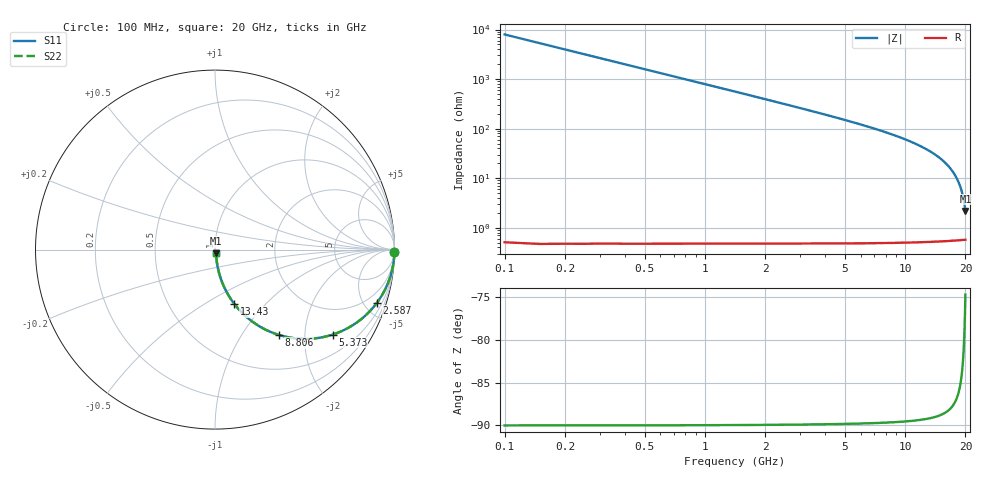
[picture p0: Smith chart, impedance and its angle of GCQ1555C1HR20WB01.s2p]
!Murata Part Number: GCQ1555C1HR20WB01
!These Parameters are Measured in Series Mode Connection
!Data Generated on Mar 13, 2026
!  o--ll--o
!Port1  Port2
!  o------o
!Operation Temp=25[degC], DC Bias Voltage=0[V]
!Freq. Start=100[MHz] Stop=20[GHz] 401[Steps]
# Hz S RI R 50
!Freq.(Hz) S11(Real) S11(Imag) S21(Real) S21(Imag) S12(Real) S12(Imag) S22(Real) S22(Imag)
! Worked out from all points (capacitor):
!   401 points, 100 MHz to 20 GHz, reference 50 ohm
!   read as one part in series: C = 200 fF near 199.5 MHz
!   lowest |Z| = 2.17 ohm at 20 GHz (marker M1)
!   S11 on the Smith chart (normalised r, x): 100 MHz: open; 2.587 GHz: 1.01, -6.05; 5.373 GHz: 1.01, -2.76; 8.806 GHz: 1.01, -1.48; 13.43 GHz: 1.01, -0.68; 20 GHz: 1.01, -0.04
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1e8  0.9998 -0.0126  0.000159 0.0126  0.000159 0.0126  0.9998 -0.0126
2.99e8  0.9986 -0.0375  0.00142 0.0375  0.00142 0.0375  0.9986 -0.0375
3.985e8  0.9975 -0.05  0.00252 0.05  0.00252 0.05  0.9975 -0.05
5.975e8  0.9944 -0.0747  0.00564 0.0747  0.00564 0.0747  0.9944 -0.0747
8.4625e8  0.9887 -0.1053  0.0113 0.1053  0.0113 0.1053  0.9887 -0.1053
1.14475e9  0.9795 -0.1413  0.0205 0.1413  0.0205 0.1413  0.9795 -0.1413
1.54275e9  0.9632 -0.1877  0.0368 0.1877  0.0368 0.1877  0.9632 -0.1877
2.04025e9  0.9369 -0.2425  0.0631 0.2425  0.0631 0.2425  0.9369 -0.2425
2.5875e9  0.9012 -0.2975  0.0988 0.2975  0.0988 0.2975  0.9012 -0.2975
3.43325e9  0.835 -0.3701  0.165 0.3701  0.165 0.3701  0.835 -0.3701
5.3735e9  0.6555 -0.4735  0.3445 0.4735  0.3445 0.4735  0.6555 -0.4735
6.7665e9  0.5243 -0.4971  0.4757 0.4971  0.4757 0.4971  0.5243 -0.4971
8.80625e9  0.3545 -0.475  0.6455 0.475  0.6455 0.475  0.3545 -0.475
1.005e10  0.2693 -0.4395  0.7307 0.4395  0.7307 0.4395  0.2693 -0.4395
1.338325e10  0.1098 -0.3052  0.8902 0.3052  0.8902 0.3052  0.1098 -0.3052
1.3433e10  0.1081 -0.303  0.8919 0.303  0.8919 0.303  0.1081 -0.303
1.5224e10  0.058 -0.2229  0.942 0.2229  0.942 0.2229  0.058 -0.2229
1.67165e10  0.0308 -0.1569  0.9692 0.1569  0.9692 0.1569  0.0308 -0.1569
1.79105e10  0.0168 -0.1056  0.9832 0.1056  0.9832 0.1056  0.0168 -0.1056
1.8806e10  0.0103 -0.0684  0.9897 0.0684  0.9897 0.0684  0.0103 -0.0684
1.945275e10  0.00744 -0.0423  0.9926 0.0423  0.9926 0.0423  0.00744 -0.0423
2e10  0.00613 -0.0207  0.9939 0.0207  0.9939 0.0207  0.00613 -0.0207
